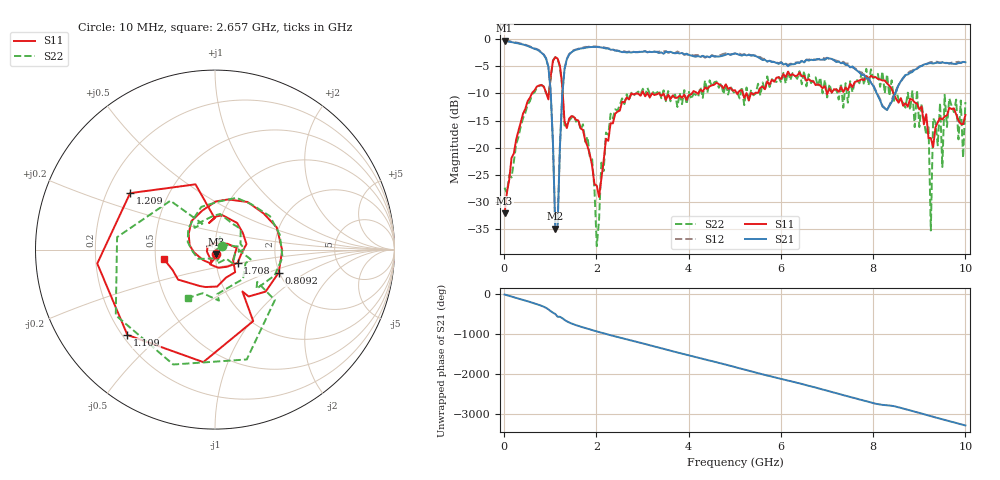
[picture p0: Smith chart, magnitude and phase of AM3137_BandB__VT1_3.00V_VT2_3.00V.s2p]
! Date/Time: Tue, Nov 13, 2018 4:52 PM
! Network Analyzer: Agilent Technologies E8364B Rev: A.07.50.67
! Sweep from 0.010 to 10.000 GHz, 201 Points, Sweep Type: LIN
! Power Supply: 3.001 V, 0.000 A
# Hz S DB R 50
!freq MagS11 AngS11 MagS21 AngS21 MagS12 AngS12 MagS22 AngS22
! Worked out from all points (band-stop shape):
!   201 points, 10 MHz to 10 GHz, reference 50 ohm
!   highest |S21| = -0.30 dB at 10 MHz (marker M1); lowest = -34.8 dB at 1.109 GHz (marker M2)
!   |S21| within 3 dB of the highest: 1.383 GHz to 4.434 GHz (3.051 GHz wide, 105 % of centre); 4.469 GHz to 5.493 GHz (1.025 GHz wide, 20.6 % of centre)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
!   lowest |S11| = -32.1 dB at 10 MHz (marker M3), VSWR 1.05, Z = 50.5 - j2.45 ohm
!   |S11| at or under -10 dB: 1.271 GHz to 2.984 GHz (1.713 GHz wide, 80.5 % of centre); 3.363 GHz to 4.07 GHz (706.9 MHz wide, 19 % of centre); 8.442 GHz to end of sweep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
!   |S22| runs from -38.1 to -3.3 dB; largest |S21 - S12| = 0.039
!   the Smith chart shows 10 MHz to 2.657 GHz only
!   S11 on the Smith chart (normalised r, x): 10 MHz: 1.01, -0.05; 809.2 MHz: 1.98, -0.60; 1.109 GHz: 0.22, -0.39; 1.209 GHz: 0.30, +0.28; 1.708 GHz: 1.27, -0.19; 2.657 GHz: 0.55, -0.06
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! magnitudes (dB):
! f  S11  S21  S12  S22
! 10 MHz  -32.1  -0.3  -0.3  -27.3
! 809.2 MHz  -8.5  -2.5  -2.4  -8.4
! 1.009 GHz  -6.9  -9.7  -9.6  -7.2
! 1.109 GHz  -3.3  -34.8  -35.1  -3.3
! 1.209 GHz  -4.9  -19.9  -19.9  -5.2
! 1.359 GHz  -16.4  -3.7  -3.7  -15.6
! 1.708 GHz  -16.7  -1.7  -1.6  -15.7
! 2.008 GHz  -26.9  -1.4  -1.4  -38.1
! 2.208 GHz  -18.3  -1.7  -1.6  -17.2
! 2.657 GHz  -10.7  -2.5  -2.4  -10.1
! 3.357 GHz  -9.9  -2.6  -2.3  -9.4
! 5.005 GHz  -9.4  -2.7  -2.6  -10.1
! 6.703 GHz  -7.8  -3.9  -3.7  -7.6
! 8.352 GHz  -8.6  -12.3  -12.2  -10.4
! 9.201 GHz  -18.2  -4.5  -4.4  -15.8
! 9.251 GHz  -18.2  -4.4  -4.2  -35.2
! 9.301 GHz  -19.9  -4.5  -4.2  -14.5
! 9.5 GHz  -14.8  -4.3  -4.3  -23.5
! 9.55 GHz  -14.2  -4.4  -4.5  -10.3
! 9.9 GHz  -15.6  -4.4  -4.3  -11.3
! 9.95 GHz  -15.7  -4.2  -4.2  -21.9
! 10 GHz  -14.0  -4.3  -4.2  -11.6
